DATA_BLOCK "TMX-DATA"
TITLE =
VERSION : 0.1


  STRUCT
   PLC_TMX : WORD ;	//Gereserveerd voor communicatie PLC --> TMX
   ControleBit : BOOL ;	//10 sec. communicatie controle bit
   StoringNiveau : BOOL ;	//Storing niveaumeting
   Hoogwatervlotter : BOOL ;	//Hoog niveau vlotter bij stilstaande pompen
   LaagNiveau : BOOL ;	//Laag niveau natte kelder
   HoogNiveau : BOOL ;	//Hoog niveau natte kelder
   StoringDebiet : BOOL ;	//Storing debietmeting
   LenspompIn : BOOL ;	//Melding lenspomp in bedrijf
   LenspompStoring : BOOL ;	//Storing lenspomp
   Pomp1Auto : BOOL ;	//Rioolwaterpomp 1 in automaat
   Pomp1Bedrijf : BOOL ;	//Rioolwaterpomp 1 in bedrijf
   Pomp1Hand : BOOL ;	//Rioolwaterpomp 1 in handbedrijf
   Pomp1NietParaat : BOOL ;	//Rioolwaterpomp 1  niet paraat
   Pomp1Storing : BOOL ;	//Rioolwaterpomp 1 in storing
   Pomp1Uit : BOOL ;	//Rioolwaterpomp 1 uit
   Pomp1WSUit : BOOL ;	//Rioolwaterpomp 1 werkschakelaar uit
   Pomp1Afsluiter1Open : BOOL ;	//Rioolwaterpomp 1 afsluiter zuig geopend
   Pomp1Afsluiter1Storing : BOOL ;	//Rioolwaterpomp 1 afsluiter zuig in storing
   Pomp2Auto : BOOL ;	//Rioolwaterpomp 2 in automaat
   Pomp2Bedrijf : BOOL ;	//Rioolwaterpomp 2 in bedrijf
   Pomp2Hand : BOOL ;	//Rioolwaterpomp 2 in handbedrijf
   Pomp2NietParaat : BOOL ;	//Rioolwaterpomp 2  niet paraat
   Pomp2Storing : BOOL ;	//Rioolwaterpomp 2 in storing
   Pomp2Uit : BOOL ;	//Rioolwaterpomp 2 uit
   Pomp2WSUit : BOOL ;	//Rioolwaterpomp 2 werkschakelaar uit
   Pomp2Afsluiter1Open : BOOL ;	//Rioolwaterpomp 2 afsluiter zuig geopend
   Pomp2Afsluiter1Storing : BOOL ;	//Rioolwaterpomp 2 afsluiter zuig in storing
   Pomp3Auto : BOOL ;	//Rioolwaterpomp 3 in automaat
   Pomp3Bedrijf : BOOL ;	//Rioolwaterpomp 3 in bedrijf
   Pomp3Hand : BOOL ;	//Rioolwaterpomp 3 in handbedrijf
   Pomp3NietParaat : BOOL ;	//Rioolwaterpomp 3  niet paraat
   Pomp3Storing : BOOL ;	//Rioolwaterpomp 3 in storing
   Pomp3Uit : BOOL ;	//Rioolwaterpomp 3 uit
   Pomp3WSUit : BOOL ;	//Rioolwaterpomp 3 werkschakelaar uit
   Pomp3AfsluiterOpen : BOOL ;	//Rioolwaterpomp 3 afsluiter zuig geopend
   Pomp3AfsluiterStoring : BOOL ;	//Rioolwaterpomp 3 afsluiter zuig in storing
   AfsluiterAf1Open : BOOL ;	//Afsluiter afgaande leiding geopend
   AfsluiterAf1Storing : BOOL ;	//Afsluiter afgaande leiding in storing
   StoringBronpomp : BOOL ;	//Bronpomp storing
   StoringVentilator : BOOL ;	//Buisventilator pompenkelder storing
   StoringHeater : BOOL ;	//Verwarming storing
   StoringNatteVentilator : BOOL ;	//Ventilator natte kelder storing
   StoringAfzuigVentilator : BOOL ;	//Ventilator afzuiging storing
   StoringBovenVentilator : BOOL ;	//MuurVentilator bovenbouw storing
   BlokkeringIn : BOOL ;	//Blokkering van gemaal actief
   GemaalParaat : BOOL ;	//Gemaal paraat
   Storing24V_alg : BOOL ;	//Storing 24V algemeen
   Storing24V_PLC_TMX : BOOL ;	//Storing 24V PLC/TMX
   Storing_UPS : BOOL ;	//Storing UPS
   StoringStroommeting : BOOL ;	//Storing stroommeting
   StoringStuurstroom : BOOL ;	//Storing stuurstroom 230V
   Overspanning : BOOL ;	//Overspanningsbeveilinging actief
   WaterOpVloer : BOOL ;	//Water op vloer alarm
   StoringkWh : BOOL ;	//Storing kWh meting
   NetspanningAfwezig : BOOL ;	//Netspanning afwezig
   VlotterNatteKelder : BOOL ;	//Vlotter in natte kelder aangesproken
   StoringAlgemeen : BOOL ;	//Verzamelstoringsmelding, lamp op kast
   Pomp1Noodbedrijf : BOOL ;	//Noodbedrijf pomp 1
   Pomp2Noodbedrijf : BOOL ;	//Noodbedrijf pomp 2
   Pomp3Noodbedrijf : BOOL ;	//Noodbedrijf pomp 3
   BlokkeringOverbrugd : BOOL ;	//Blokkering van gemaal lokaal op TP overbrugd
   StuurstroomMotoren : BOOL ;	//Storing stuurstroom motorgroepen
   StuurstroomMetingen : BOOL ;	//Storing Stuurstroom metingen
   StuurstroomHWvlotter : BOOL ;	//Storing Stuurstroom hoogwatervlotter
   AfsluiterDicht : BOOL ;	//Afsluiter afgaande leiding gesloten
   Pomp1Afsluiter1Dicht : BOOL ;	//Rioolwaterpomp 1 afsluiter zuig gesloten
   Pomp2Afsluiter1Dicht : BOOL ;	//Rioolwaterpomp 2 afsluiter zuig gesloten
   Pomp3fsluiter1Dicht : BOOL ;	//Rioolwaterpomp 3 afsluiter zuig gesloten
   Pomp1Afsluiter2Storing : BOOL ;	//Rioolwaterpomp 1 afsluiter pers in storing
   Pomp1Afsluiter2Open : BOOL ;	//Rioolwaterpomp 1 afsluiter pers in open
   Pomp1Afsluiter2Dicht : BOOL ;	//Rioolwaterpomp 1 afsluiter pers gesloten
   Pomp2Afsluiter2Storing : BOOL ;	//Rioolwaterpomp 2 afsluiter pers in storing
   Pomp2Afsluiter2Open : BOOL ;	//Rioolwaterpomp 2 afsluiter pers geopend
   Pomp2Afsluiter2Dicht : BOOL ;	//Rioolwaterpomp 2 afsluiter pers gesloten
   Pomp3Afsluiter2Storing : BOOL ;	//Rioolwaterpomp 3 afsluiter pers in storing
   Pomp3Afsluiter2Open : BOOL ;	//Rioolwaterpomp 3 afsluiter pers geopend
   Pomp3Afsluiter2Dicht : BOOL ;	//Rioolwaterpomp 3 afsluiter pers gesloten
   StoringHydrofoor : BOOL ;	//Hydrofoorset storing
   AfsluiterAf1Dicht : BOOL ;	//Afsluiter afgaande persleiding 1 dicht
   AfsluiterAf2Storing : BOOL ;	//Afsluiter afgaande persleiding 2 storing
   AfsluiterAf2Open : BOOL ;	//Afsluiter afgaande persleiding 2 geopend
   AfsluiterAf2Dicht : BOOL ;	//Afsluiter afgaande persleiding 2 dicht
   AfsluiterBypStoring : BOOL ;	//Afsluiter Bijpass storing
   AfsluiterBypOpen : BOOL ;	//Afsluiter Bijpass open
   AfsluiterBypDicht : BOOL ;	//Afsluiter Bijpass dicht
   AfsluiterPigStoring : BOOL ;	//Afsluiter Piglancering persleiding 1 storing
   AfsluiterPigOpen : BOOL ;	//Afsluiter Piglancering persleiding 1 open
   AfsluiterPigDicht : BOOL ;	//Afsluiter Piglancering persleiding 1 dicht
   ReserveBit12_7 : BOOL ;	//reserve
   ReserveBit13_0 : BOOL ;	//reserve
   ReserveBit13_1 : BOOL ;	//reserve
   ReserveBit13_2 : BOOL ;	//reserve
   ReserveBit13_3 : BOOL ;	//reserve
   ReserveBit13_4 : BOOL ;	//reserve
   Inslagpeil : INT ;	//Inslagpeil, niveau start pompen
   Uitslagpeil : INT ;	//Uitslagpeil, niveau stop pompen
   Debiet : INT ;	//Debietmeting
   Stroom : INT ;	//Stroommeting gemaal
   Pomp1Toerental : INT ;	//Actueel toerental rioolwaterpomp 1
   Pomp2Toerental : INT ;	//Actueel toerental rioolwaterpomp 2
   Pomp3Toerental : INT ;	//Actueel toerental rioolwaterpomp 3
   DebietTeller : INT ;	//Totaal debiet in m3
   KwhTeller : INT ;	//Totaal Kwh teller in Kwh
   Niveau : INT ;	//Niveaumeting
   NiveauStuwput : INT ;	//Niveaumeting stuwput
   Pomp1Stoom : INT ;	//Actueel stroom rioolwaterpomp 1
   Pomp2Stoom : INT ;	//Actueel stroom rioolwaterpomp 2
   Pomp3Stoom : INT ;	//Actueel stroom rioolwaterpomp 3
   Reservebyte42 : BYTE ;
   Reservebyte43 : BYTE ;
   Reservebyte44 : BYTE ;
   Reservebyte45 : BYTE ;
   Reservebyte46 : BYTE ;
   Reservebyte47 : BYTE ;
   Reservebyte48 : BYTE ;
   Reservebyte49 : BYTE ;
   TMX_PLC : WORD ;	//Gereserveer voor communicatie TMX --> PLC
   BlokkeringTMX : BOOL ;	//Blokkeringsaanvraag van TMX
   ResetTMX : BOOL ;	//Reset alarm van TMX, opgaande flank
   ReserveTMX1 : WORD ;	//reserve
   ReserveTMX2 : WORD ;	//reserve
   ReserveTMX3 : WORD ;	//reserve
   ReserveTMX4 : WORD ;	//reserve
   ReserveTMX5 : WORD ;	//reserve
  END_STRUCT ;
BEGIN
   PLC_TMX := W#16#0;
   ControleBit := FALSE;
   StoringNiveau := FALSE;
   Hoogwatervlotter := FALSE;
   LaagNiveau := FALSE;
   HoogNiveau := FALSE;
   StoringDebiet := FALSE;
   LenspompIn := FALSE;
   LenspompStoring := FALSE;
   Pomp1Auto := FALSE;
   Pomp1Bedrijf := FALSE;
   Pomp1Hand := FALSE;
   Pomp1NietParaat := FALSE;
   Pomp1Storing := FALSE;
   Pomp1Uit := FALSE;
   Pomp1WSUit := FALSE;
   Pomp1Afsluiter1Open := FALSE;
   Pomp1Afsluiter1Storing := FALSE;
   Pomp2Auto := FALSE;
   Pomp2Bedrijf := FALSE;
   Pomp2Hand := FALSE;
   Pomp2NietParaat := FALSE;
   Pomp2Storing := FALSE;
   Pomp2Uit := FALSE;
   Pomp2WSUit := FALSE;
   Pomp2Afsluiter1Open := FALSE;
   Pomp2Afsluiter1Storing := FALSE;
   Pomp3Auto := FALSE;
   Pomp3Bedrijf := FALSE;
   Pomp3Hand := FALSE;
   Pomp3NietParaat := FALSE;
   Pomp3Storing := FALSE;
   Pomp3Uit := FALSE;
   Pomp3WSUit := FALSE;
   Pomp3AfsluiterOpen := FALSE;
   Pomp3AfsluiterStoring := FALSE;
   AfsluiterAf1Open := FALSE;
   AfsluiterAf1Storing := FALSE;
   StoringBronpomp := FALSE;
   StoringVentilator := FALSE;
   StoringHeater := FALSE;
   StoringNatteVentilator := FALSE;
   StoringAfzuigVentilator := FALSE;
   StoringBovenVentilator := FALSE;
   BlokkeringIn := FALSE;
   GemaalParaat := FALSE;
   Storing24V_alg := FALSE;
   Storing24V_PLC_TMX := FALSE;
   Storing_UPS := FALSE;
   StoringStroommeting := FALSE;
   StoringStuurstroom := FALSE;
   Overspanning := FALSE;
   WaterOpVloer := FALSE;
   StoringkWh := FALSE;
   NetspanningAfwezig := FALSE;
   VlotterNatteKelder := FALSE;
   StoringAlgemeen := FALSE;
   Pomp1Noodbedrijf := FALSE;
   Pomp2Noodbedrijf := FALSE;
   Pomp3Noodbedrijf := FALSE;
   BlokkeringOverbrugd := FALSE;
   StuurstroomMotoren := FALSE;
   StuurstroomMetingen := FALSE;
   StuurstroomHWvlotter := FALSE;
   AfsluiterDicht := FALSE;
   Pomp1Afsluiter1Dicht := FALSE;
   Pomp2Afsluiter1Dicht := FALSE;
   Pomp3fsluiter1Dicht := FALSE;
   Pomp1Afsluiter2Storing := FALSE;
   Pomp1Afsluiter2Open := FALSE;
   Pomp1Afsluiter2Dicht := FALSE;
   Pomp2Afsluiter2Storing := FALSE;
   Pomp2Afsluiter2Open := FALSE;
   Pomp2Afsluiter2Dicht := FALSE;
   Pomp3Afsluiter2Storing := FALSE;
   Pomp3Afsluiter2Open := FALSE;
   Pomp3Afsluiter2Dicht := FALSE;
   StoringHydrofoor := FALSE;
   AfsluiterAf1Dicht := FALSE;
   AfsluiterAf2Storing := FALSE;
   AfsluiterAf2Open := FALSE;
   AfsluiterAf2Dicht := FALSE;
   AfsluiterBypStoring := FALSE;
   AfsluiterBypOpen := FALSE;
   AfsluiterBypDicht := FALSE;
   AfsluiterPigStoring := FALSE;
   AfsluiterPigOpen := FALSE;
   AfsluiterPigDicht := FALSE;
   ReserveBit12_7 := FALSE;
   ReserveBit13_0 := FALSE;
   ReserveBit13_1 := FALSE;
   ReserveBit13_2 := FALSE;
   ReserveBit13_3 := FALSE;
   ReserveBit13_4 := FALSE;
   Inslagpeil := 0;
   Uitslagpeil := 0;
   Debiet := 0;
   Stroom := 0;
   Pomp1Toerental := 0;
   Pomp2Toerental := 0;
   Pomp3Toerental := 0;
   DebietTeller := 0;
   KwhTeller := 0;
   Niveau := 0;
   NiveauStuwput := 0;
   Pomp1Stoom := 0;
   Pomp2Stoom := 0;
   Pomp3Stoom := 0;
   Reservebyte42 := B#16#0;
   Reservebyte43 := B#16#0;
   Reservebyte44 := B#16#0;
   Reservebyte45 := B#16#0;
   Reservebyte46 := B#16#0;
   Reservebyte47 := B#16#0;
   Reservebyte48 := B#16#0;
   Reservebyte49 := B#16#0;
   TMX_PLC := W#16#0;
   BlokkeringTMX := FALSE;
   ResetTMX := FALSE;
   ReserveTMX1 := W#16#0;
   ReserveTMX2 := W#16#0;
   ReserveTMX3 := W#16#0;
   ReserveTMX4 := W#16#0;
   ReserveTMX5 := W#16#0;
END_DATA_BLOCK

